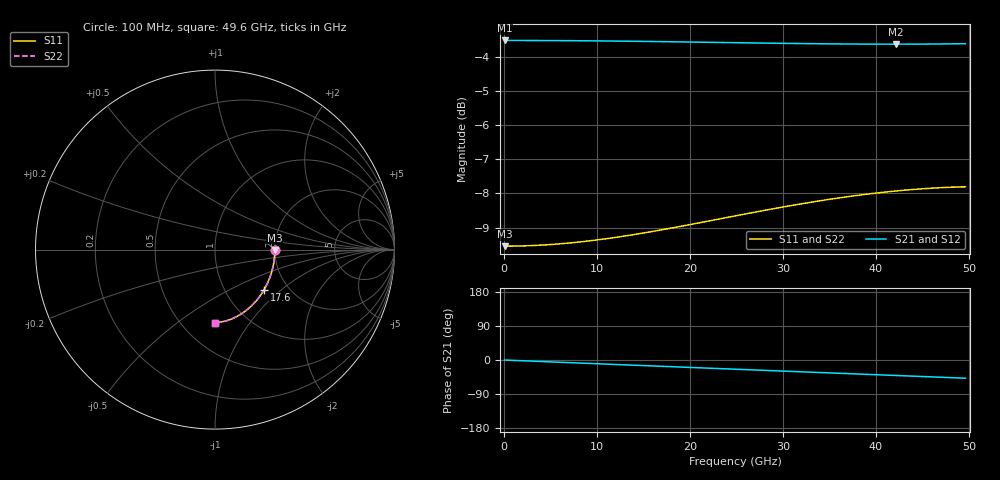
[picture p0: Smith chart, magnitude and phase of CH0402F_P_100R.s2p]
# GHz S RI R 100
! S-Parameters data
! Freq  reS11  imS11  reS21  imS21  reS12  imS12  reS22  imS22
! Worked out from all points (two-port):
!   100 points, 100 MHz to 49.6 GHz, reference 100 ohm
!   highest |S21| = -3.52 dB at 100 MHz (marker M1); lowest = -3.6 dB at 42.1 GHz (marker M2)
!   |S21| within 3 dB of the highest: start of sweep to end of sweep
!   lowest |S11| = -9.5 dB at 100 MHz (marker M3), VSWR 2.00, Z = 200 - j0.616 ohm
!   |S11| at or under -10 dB: nowhere
!   |S22| runs from -9.5 to -7.8 dB; largest |S21 - S12| = 0
!   S11 on the Smith chart (normalised r, x): 100 MHz: 2.00, -0.01; 17.6 GHz: 1.51, -0.78; 49.6 GHz: 0.72, -0.70
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0.1  0.3333 -0.00137  0.6667 -0.00114  0.6667 -0.00114  0.3333 -0.00137
2.1  0.3324 -0.0287  0.6662 -0.024  0.6662 -0.024  0.3324 -0.0287
4.1  0.3299 -0.0559  0.6648 -0.0469  0.6648 -0.0469  0.3299 -0.0559
6.1  0.3257 -0.0828  0.6626 -0.0696  0.6626 -0.0696  0.3257 -0.0828
8.6  0.3182 -0.1157  0.6587 -0.0979  0.6587 -0.0979  0.3182 -0.1157
10.6  0.3105 -0.1414  0.6546 -0.1203  0.6546 -0.1203  0.3105 -0.1414
12.6  0.3014 -0.1664  0.6497 -0.1425  0.6497 -0.1425  0.3014 -0.1664
16.6  0.2791 -0.2136  0.6375 -0.1862  0.6375 -0.1862  0.2791 -0.2136
17.6  0.2727 -0.2248  0.634 -0.1969  0.634 -0.1969  0.2727 -0.2248
21.6  0.2447 -0.2667  0.6181 -0.239  0.6181 -0.239  0.2447 -0.2667
25.1  0.2171 -0.2992  0.6019 -0.2746  0.6019 -0.2746  0.2171 -0.2992
27.1  0.2003 -0.3159  0.5918 -0.2944  0.5918 -0.2944  0.2003 -0.3159
29.1  0.183 -0.3312  0.5811 -0.3139  0.5811 -0.3139  0.183 -0.3312
31.1  0.1652 -0.3452  0.5698 -0.3329  0.5698 -0.3329  0.1652 -0.3452
33.1  0.1471 -0.3577  0.5579 -0.3515  0.5579 -0.3515  0.1471 -0.3577
35.1  0.1287 -0.3687  0.5455 -0.3698  0.5455 -0.3698  0.1287 -0.3687
37.1  0.1103 -0.3783  0.5326 -0.3876  0.5326 -0.3876  0.1103 -0.3783
39.1  0.0919 -0.3865  0.5192 -0.4051  0.5192 -0.4051  0.0919 -0.3865
41.6  0.069 -0.3948  0.5017 -0.4263  0.5017 -0.4263  0.069 -0.3948
42.1  0.0645 -0.3962  0.4981 -0.4305  0.4981 -0.4305  0.0645 -0.3962
45.6  0.0334 -0.4036  0.4722 -0.4592  0.4722 -0.4592  0.0334 -0.4036
49.6  -0.000254 -0.4072  0.4407 -0.4906  0.4407 -0.4906  -0.000254 -0.4072
